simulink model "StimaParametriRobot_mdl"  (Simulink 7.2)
settings: Solver=ode3  StartTime=0.0  StopTime=Tf  FixedStep=dt  RelTol=1e-3
undefined symbols (not defined in the file or in its folder): DinamicaInversaRobot2gdl

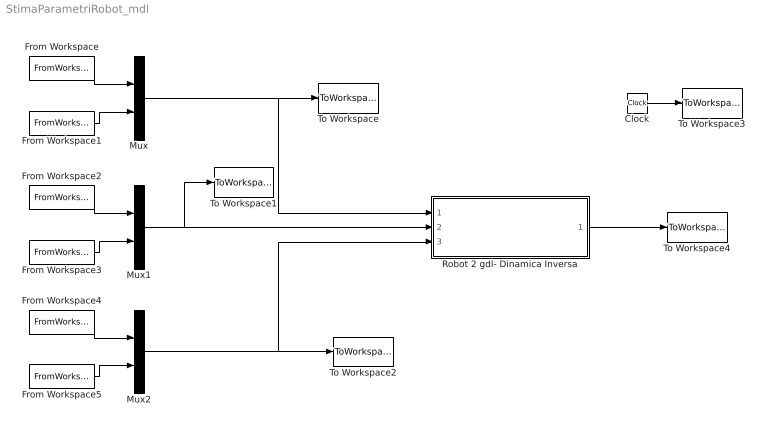
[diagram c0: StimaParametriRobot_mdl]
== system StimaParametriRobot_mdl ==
  Clock : Clock
  From Workspace : FromWorkspace  VariableName=[time' q1']  SampleTime=0
  From Workspace1 : FromWorkspace  VariableName=[time' q2']  SampleTime=0
  From Workspace2 : FromWorkspace  VariableName=[time' dq1']  SampleTime=0
  From Workspace3 : FromWorkspace  VariableName=[time' dq2']  SampleTime=0
  From Workspace4 : FromWorkspace  VariableName=[time' ddq1']  SampleTime=0
  From Workspace5 : FromWorkspace  VariableName=[time' ddq2']  SampleTime=0
  Mux : Mux  Inputs=2
  Mux1 : Mux  Inputs=2
  Mux2 : Mux  Inputs=2
  Robot 2 gdl- Dinamica Inversa : Subsystem
  To Workspace : ToWorkspace  VariableName=Q  SampleTime=-1  SaveFormat=Array
  To Workspace1 : ToWorkspace  VariableName=DQ  SampleTime=-1  SaveFormat=Array
  To Workspace2 : ToWorkspace  VariableName=DDQ  SampleTime=-1  SaveFormat=Array
  To Workspace3 : ToWorkspace  VariableName=times  SampleTime=-1  SaveFormat=Array
  To Workspace4 : ToWorkspace  VariableName=Tau  SampleTime=-1  SaveFormat=Array
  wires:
  Robot 2 gdl- Dinamica Inversa/1(tau) -> To Workspace4/1
  From Workspace/1 -> Mux/1
  From Workspace1/1 -> Mux/2
  From Workspace2/1 -> Mux1/1
  From Workspace3/1 -> Mux1/2
  From Workspace4/1 -> Mux2/1
  From Workspace5/1 -> Mux2/2
  Mux/1 -> Robot 2 gdl- Dinamica Inversa/1(q), To Workspace/1
  Mux1/1 -> Robot 2 gdl- Dinamica Inversa/2(dq), To Workspace1/1
  Mux2/1 -> Robot 2 gdl- Dinamica Inversa/3(ddq), To Workspace2/1
  Clock/1 -> To Workspace3/1

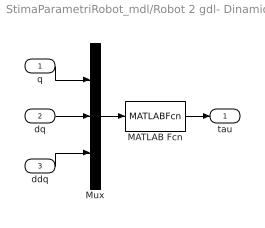
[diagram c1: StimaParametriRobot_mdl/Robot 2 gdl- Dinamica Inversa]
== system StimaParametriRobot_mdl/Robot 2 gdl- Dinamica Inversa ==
  q : Inport
  dq : Inport  Port=2
  ddq : Inport  Port=3
  MATLAB Fcn : MATLABFcn  MATLABFcn="DinamicaInversaRobot2gdl([u(1)  u(2)]',[u(3)  u(4)]',[u(5)  u(6)]')"  OutputDimensions=2
  Mux : Mux  Inputs=3
  tau : Outport
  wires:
  Mux/1 -> MATLAB Fcn/1
  dq/1 -> Mux/2
  ddq/1 -> Mux/3
  MATLAB Fcn/1 -> tau/1
  q/1 -> Mux/1
